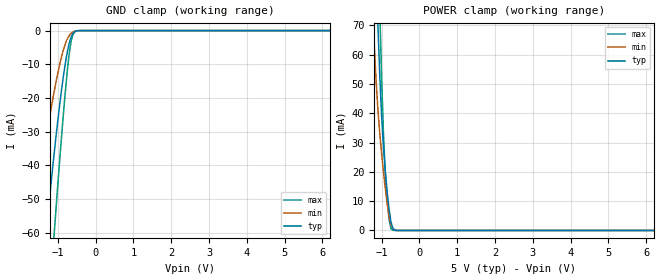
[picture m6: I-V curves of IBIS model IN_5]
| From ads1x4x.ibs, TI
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|   INPUT 5.0V Model
[Model]   IN_5
Model_type   Input
| Signals   nRESET, START, nCS, DIN, SCLK
Vinl = 0.75V
Vinh = 2.00V
| variable   typ   min   max
C_comp   6.377pF   7.107pF   5.764pF
[Temperature Range]   40.0   105.0   -40.0
[Voltage range]   5.0V   4.75V   5.25V
[power clamp reference] 5.0V   4.75V   5.25V
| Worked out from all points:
|   GND clamp passes 1 mA (typ) near -0.61 V on its own axis
|   POWER clamp passes 1 mA (typ) near -0.71 V on its own axis
[GND Clamp]
|   Voltage   I(typ)   I(min)   I(max)
-5V       -567.5mA   -418.5mA   -701.3mA
-1.65V    -102.4mA   -59.28mA   -150mA
-1.3V     -59.09mA   -31.55mA   -92.59mA
-1.1V     -36.8mA    -18.29mA   -60.87mA
-1.05V    -31.64mA   -15.34mA   -53.2mA
-900mV    -17.48mA   -7.66mA    -31.25mA
-750mV    -6.367mA   -2.478mA   -12.03mA
-700mV    -3.772mA   -1.484mA   -6.955mA
-650mV    -1.918mA   -829.5uA   -3.262mA
-600mV    -803.4uA   -434.9uA   -1.177mA
-550mV    -277.7uA   -212uA     -329.4uA
10V       0A         0A         0A
[POWER Clamp]
|   Voltage   I(typ)   I(min)   I(max)
-5V       2.152A     1.797A     2.717A
-1.25V    136.5mA    80.6mA     194.5mA
-1.2V     113.4mA    65.19mA    163.6mA
-1.1V     71.21mA    41.78mA    104.4mA
-1.05V    53.46mA    33.45mA    77mA
-1V       39.14mA    26.36mA    52.5mA
-950mV    28.36mA    19.98mA    32.82mA
-900mV    19.98mA    14.14mA    19.24mA
-850mV    12.96mA    8.929mA    9.991mA
-800mV    7.072mA    4.678mA    3.559mA
-700mV    700.2uA    550.5uA    59.14uA
10V       0A         0A         0A
